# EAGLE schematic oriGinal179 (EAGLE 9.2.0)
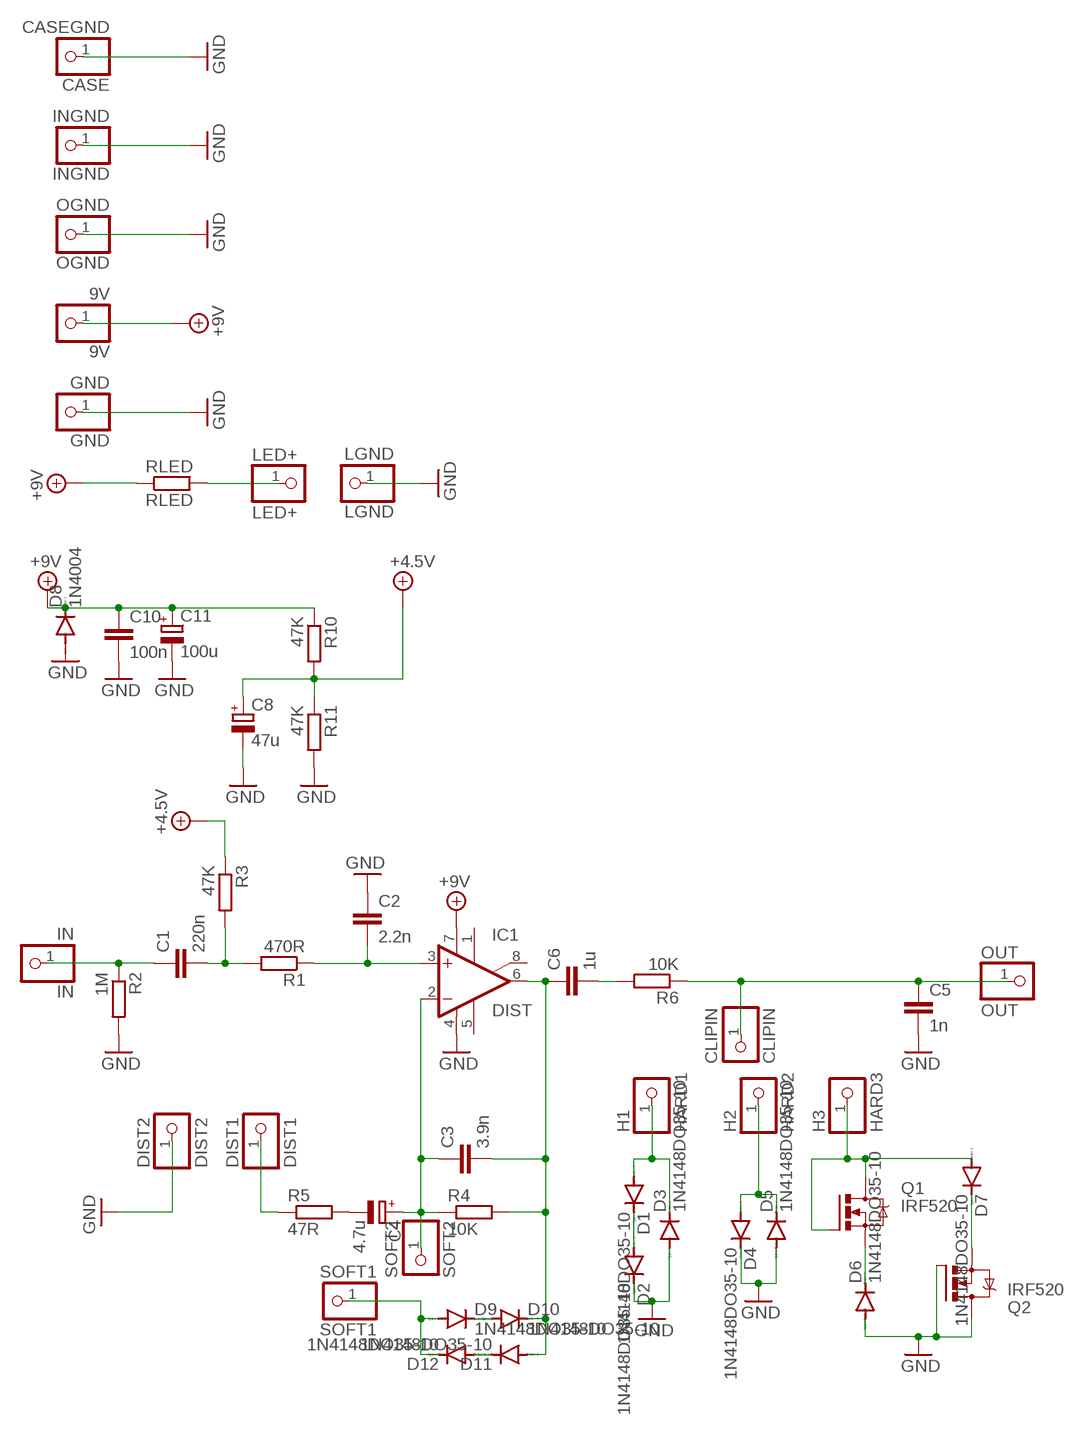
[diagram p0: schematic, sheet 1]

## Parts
9V  9V  PINHD-1X1  [1X01]
C1  220n  C5/7.2  [C5B7.2]
C2  2.2n  C5/5.5  [C5B5.5]
C3  3.9n  C-EU075-052X106  [C075-052X106]
C4  4.7u  CPOL-EUE15-5AXIAL  [E15-5]
C5  1n  C5/7.2  [C5B7.2]
C6  1u  C-EU150-084X183  [C150-084X183]
C8  47u  CPOL-EUE15-9AXIAL  [E15-9]
C10  100n  C5/7.2  [C5B7.2]
C11  100u  CPOL-EUE22-9AXIAL  [E22-9]
CASE  CASEGND  PINHD-1X1  [1X01]
CLIPIN  CLIPIN  PINHD-1X1  [1X01]
D1  1N4148DO35-10  [DO35-10]
D2  1N4148DO35-10  [DO35-10]
D3  1N4148DO35-10  [DO35-10]
D4  1N4148DO35-10  [DO35-10]
D5  1N4148DO35-10  [DO35-10]
D6  1N4148DO35-10  [DO35-10]
D7  1N4148DO35-10  [DO35-10]
D8  1N4004  [DO41-10]
D9  1N4148DO35-10  [DO35-10]
D10  1N4148DO35-10  [DO35-10]
D11  1N4148DO35-10  [DO35-10]
D12  1N4148DO35-10  [DO35-10]
DIST1  DIST1  PINHD-1X1  [1X01]
DIST2  DIST2  PINHD-1X1  [1X01]
GND  GND  PINHD-1X1  [1X01]
H1  HARD1  PINHD-1X1  [1X01]
H2  HARD2  PINHD-1X1  [1X01]
H3  HARD3  PINHD-1X1  [1X01]
IC1  DIST  NE5534AN  [DIL08]
IN  IN  PINHD-1X1  [1X01]
INGND  INGND  PINHD-1X1  [1X01]
LED+  LED+  PINHD-1X1  [1X01]
LGND  LGND  PINHD-1X1  [1X01]
OGND  OGND  PINHD-1X1  [1X01]
OUT  OUT  PINHD-1X1  [1X01]
Q1  IRF520  [TO220BV]
Q2  IRF520  [TO220BV]
R1  470R  R-EU_0207/10  [0207/10]
R2  1M  R-EU_0207/10  [0207/10]
R3  47K  R-EU_0207/10  [0207/10]
R4  10K  R-EU_0207/10  [0207/10]
R5  47R  R-EU_0207/10  [0207/10]
R6  10K  R-EU_0207/10  [0207/10]
R10  47K  R-EU_0207/10  [0207/10]
R11  47K  R-EU_0207/10  [0207/10]
RLED  RLED  R-EU_0207/10  [0207/10]
SOFT1  SOFT1  PINHD-1X1  [1X01]
SOFT2  SOFT2  PINHD-1X1  [1X01]

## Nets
+4.1V: C8.+ R3.1 R10.2 R11.1 ; supply symbol labelled +4.5V
+12V: 9V.1 C10.1 C11.+ D8.C IC1.7(V+) R10.1 RLED.1 ; supply symbol labelled +9V
GND [GND]: C2.1 C5.2 C8.- C10.2 C11.- CASE.1 D2.C D3.A D4.C D5.A D6.A D8.A DIST2.1 GND.1 IC1.4(V-) INGND.1 LGND.1 OGND.1 Q2.D Q2.G R2.2 R11.2
H3: D7.A H3.1 Q1.D Q1.G
N$1: C1.1 IN.1 R2.1
N$2: C1.2 R1.2 R3.2
N$3: C2.2 IC1.3(+IN) R1.1
N$4: C4.- R5.2
N$5: C3.1 C4.+ IC1.2(-IN) R4.1 SOFT2.1
N$6: D9.A D12.C SOFT1.1
N$7: DIST1.1 R5.1
N$8: C5.1 CLIPIN.1 OUT.1 R6.1
N$9: D6.C Q1.S
N$11: D11.C D12.A
N$12: D7.C Q2.S
N$13: D4.A D5.C H2.1
N$14: D9.C D10.A
N$16: D1.C D2.A
N$17: D1.A D3.C H1.1
N$19: C3.2 C6.1 D10.C D11.A IC1.6(OUT) R4.2
N$20: LED+.1 RLED.2
N$21: C6.2 R6.2
Unconnected: IC1.1(ON) IC1.5(CMP) IC1.8(ON/CMP)

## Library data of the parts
9V CASE CLIPIN DIST1 DIST2 GND H1-H3 IN INGND LED+ LGND OGND OUT SOFT1 SOFT2 = pinhead:PINHD-1X1: PIN HEADER
C1 C2 C5 C10 = capacitor-wima:C: CAPACITOR
C3 C6 = rcl:C-EU: CAPACITOR, European symbol; SPICEPREFIX: C
C4 C8 C11 = rcl:CPOL-EU: POLARIZED CAPACITOR, European symbol; SPICEPREFIX: C
D1-D7 D9-D12 = diode:1N4148: DIODE
D8 = diode:1N4004: DIODE
IC1 = linear:NE5534: LOW-NOISE OPERATIONAL AMPLIFIER Source: http://focus.ti.com/lit/ds/symlink/ne5534.pdf
Q1 Q2 = transistor-power:IRF520: HEXFET Power MOSFET
R1-R6 R10 R11 RLED = rcl:R-EU_: RESISTOR, European symbol; SPICEPREFIX: R

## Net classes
0 default: width 0.406 mm, drill 0.032 mm
1 GND: width 24 mm, drill 0.032 mm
